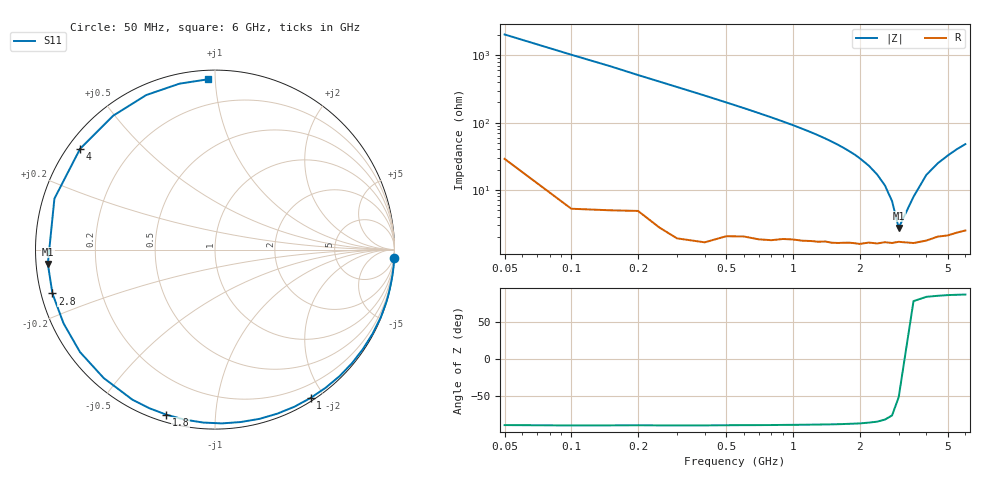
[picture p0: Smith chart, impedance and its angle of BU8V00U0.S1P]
! Infineon Technologies  Discrete & RF Semiconductors
! BB 833
! Si Tuning Diode in SOD323
! VR = 8 V
! S-Parameters:  June  1999
# GHz  S  MA  R  50
!  f  S11
! GHz  MAG  ANG
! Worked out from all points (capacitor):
!   34 points, 50 MHz to 6 GHz, reference 50 ohm
!   read as one part to ground: C = 1.56 pF near 50 MHz
!   lowest |Z| = 2.72 ohm at 3 GHz (marker M1)
!   series resonance near 3.108 GHz, so ESL is about 1.7 nH
!   S11 on the Smith chart (normalised r, x): 50 MHz: 1, -41; 1 GHz: 0.04, -1.83; 1.8 GHz: 0.03, -0.75; 2.8 GHz: 0.03, -0.13; 4 GHz: 0.04, +0.33; 6 GHz: 0.05, +0.96
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0.05  0.9993 -2.8
0.15  0.999 -8.3
0.25  0.9984 -14.0
0.4  0.9975 -22.4
0.6  0.9932 -33.8
0.8  0.9894 -45.4
1  0.9834 -57.2
1.1  0.9809 -63.2
1.2  0.9778 -69.2
1.3  0.975 -75.3
1.4  0.9713 -81.5
1.5  0.9691 -87.7
1.6  0.9659 -93.9
1.7  0.9622 -100.2
1.8  0.9588 -106.4
1.9  0.9565 -112.5
2  0.9545 -118.8
2.2  0.947 -130.9
2.4  0.9443 -142.8
2.6  0.9387 -154.0
2.8  0.9382 -164.9
3  0.9348 -175.1
3.5  0.9387 162.4
4  0.9385 143.2
4.5  0.9373 127.3
5  0.9425 114.0
5.5  0.9454 102.1
6  0.9493 92.5
